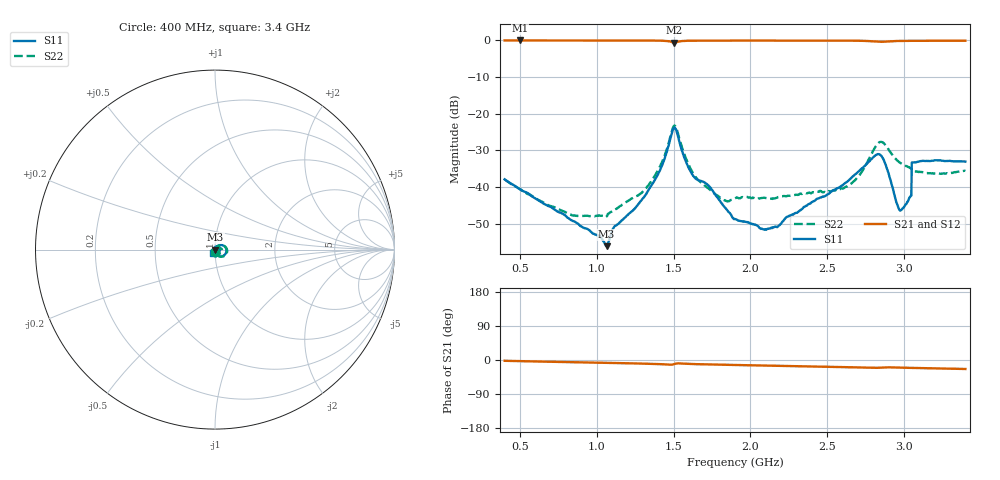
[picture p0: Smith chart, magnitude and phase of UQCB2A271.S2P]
!  Part Number  UQCB2A271	Mounting Orientation: Vertical
!  Description: RF capacitors
!  Application: Coupling, Bypass, Tuning, DC Block
!  Filters, Matching
# GHZ S DB R 50
! Freq  |S11|  S11 Ph  |S21|  S21 Ph  |S12|  S12 Ph  |S22|  S22 Ph
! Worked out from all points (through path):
!   801 points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, 400 MHz to 3.4 GHz, reference 50 ohm
!   highest |S21| = -0.02 dB at 501 MHz (marker M1); lowest = -0.6 dB at 1.506 GHz (marker M2)
!   group delay of S21, straight-line fit = 19.6 ps
!   lowest |S11| = -56.2 dB at 1.064 GHz (marker M3), VSWR 1.00, Z = 50.2 + j0.036 ohm
!   |S11| at or under -10 dB: start of sweep to end of sweep
!   |S22| runs from -48.2 to -23.2 dB; largest |S21 - S12| = 0.0035
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0.4  -37.92 -79.9  -0.02 -2.1  -0.04 -2.1  -37.94 -78.4
0.501  -40.68 -76.2  -0.02 -3.0  -0.04 -3.0  -40.59 -72.9
0.903  -50.88 -40.4  -0.03 -6.3  -0.05 -6.2  -47.92 -23.5
1.064  -56.16 13.3  -0.04 -7.5  -0.06 -7.5  -48.04 12.3
1.116  -50.74 38.4  -0.04 -7.9  -0.06 -7.9  -46.33 19.5
1.293  -43.54 61.6  -0.04 -9.5  -0.06 -9.4  -41.59 41.3
1.401  -36.32 61.8  -0.07 -10.7  -0.09 -10.7  -35.22 50.0
1.506  -23.81 -11.2  -0.62 -10.6  -0.63 -10.6  -23.25 -12.0
1.596  -34.60 -79.7  -0.09 -10.2  -0.11 -10.2  -33.74 -73.7
1.656  -38.08 -80.5  -0.07 -11.1  -0.08 -11.0  -37.92 -70.0
1.836  -45.70 -119.0  -0.06 -12.6  -0.08 -12.6  -43.68 -47.5
1.9  -48.76 -120.5  -0.05 -13.1  -0.07 -13.1  -43.16 -36.2
2.118  -51.33 -167.2  -0.05 -14.9  -0.07 -14.8  -43.16 -27.9
2.403  -44.09 131.6  -0.06 -17.1  -0.08 -17.1  -41.48 -11.4
2.643  -38.10 94.6  -0.08 -19.1  -0.10 -19.0  -39.44 12.4
2.826  -31.08 15.8  -0.35 -20.6  -0.37 -20.6  -28.33 2.1
2.901  -36.51 -65.4  -0.26 -19.4  -0.28 -19.3  -29.90 -42.4
2.961  -45.37 -135.1  -0.16 -20.0  -0.17 -19.9  -32.99 -45.0
2.984  -46.19 -169.2  -0.14 -20.2  -0.16 -20.2  -33.65 -42.9
3.033  -43.23 140.9  -0.13 -20.7  -0.14 -20.7  -34.60 -38.1
3.066  -33.29 -96.5  -0.11 -21.0  -0.13 -20.9  -35.65 -90.6
3.4  -33.07 -114.2  -0.09 -23.7  -0.10 -23.7  -35.63 -105.4
